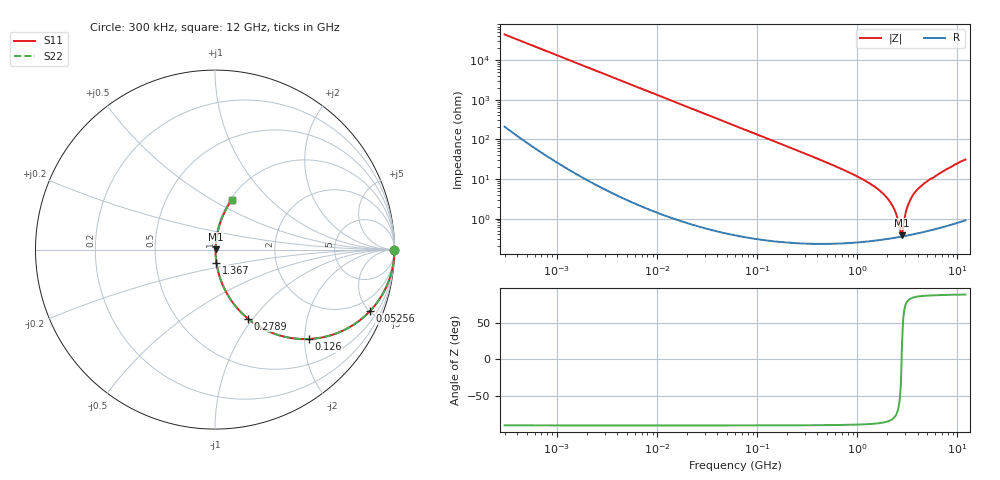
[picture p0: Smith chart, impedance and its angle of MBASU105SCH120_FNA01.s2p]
! MBASU105SCH120_FNA01  S-PARAMETER MODEL  ( General Type )
! Model Generated by TAIYO YUDEN Corporation (http://www.ty-top.com)
! Version 1.0
! TAIYO YUDEN Control No. 130207
! Copyright(c) 2013 TAIYO YUDEN CO.,LTD. All Rights Reserved.
! Product Description (link to TY-COMPAS)
! https://ds.yuden.co.jp/TYCOMPAS/or/detail?pn=MBASU105SCH120JFNA01&u=M
! Products Name : Multilayer Ceramic Capacitors
! Characteristics :
!  Capacitance : 12 pF , Rated Voltage : 50V , TCC : CH / C0H
!  Case Size : 1.0 x 0.5 / 0.039 x 0.02 [mm/inch] , Thickness : 0.5 / 0.02 [mm/inch]
!  (Conditions: Temperature = 25 degC , DC Bias Current/Voltage = 0A / 0V)
! External Node Assignments :
!  1  o---| |---o  2
! GND o---------o GND
! Frequency Range : 300000Hz  -  12GHz  [ 401 STEP ]
# MHz S RI R 50
! Freq[MHz].  S11 Real  S11 Imag  S21 Real  S21 Imag  S12 Real  S12 Imag  S22 Real  S22 Imag
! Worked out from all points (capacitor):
!   401 points, 300 kHz to 12 GHz, reference 50 ohm
!   read as one part in series: C = 12 pF near 316.3 kHz
!   lowest |Z| = 382 mohm at 2.795 GHz (marker M1)
!   series resonance near 2.768 GHz, so ESL is about 280 pH
!   S11 on the Smith chart (normalised r, x): 300 kHz: open; 52.56 MHz: 1.01, -5.05; 126 MHz: 1.01, -2.10; 278.9 MHz: 1.00, -0.94; 1.367 GHz: 1.01, -0.15; 12 GHz: 1.02, +0.62
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0.3  1 -0.00226  1.57e-05 0.00226  1.57e-05 0.00226  1 -0.00226
1.769972  0.9998 -0.0133  0.000197 0.0133  0.000197 0.0133  0.9998 -0.0133
10.44266  0.9938 -0.0782  0.00623 0.0782  0.00623 0.0782  0.9938 -0.0782
27.82928  0.9577 -0.2007  0.0423 0.2007  0.0423 0.2007  0.9577 -0.2007
52.55639  0.864 -0.342  0.136 0.342  0.136 0.342  0.864 -0.342
60  0.8298 -0.3749  0.1702 0.3749  0.1702 0.3749  0.8298 -0.3749
125.9782  0.5251 -0.498  0.4749 0.498  0.4749 0.498  0.5251 -0.498
278.9009  0.1829 -0.3841  0.8171 0.3841  0.8171 0.3841  0.1829 -0.3841
353.9943  0.1214 -0.3234  0.8786 0.3234  0.8786 0.3234  0.1214 -0.3234
783.7017  0.026 -0.1516  0.974 0.1516  0.974 0.1516  0.026 -0.1516
1366.97  0.00807 -0.073  0.9919 0.073  0.9919 0.073  0.00807 -0.073
1735.023  0.00508 -0.0465  0.9949 0.0465  0.9949 0.0465  0.00508 -0.0465
2088.533  0.00388 -0.0277  0.9961 0.0277  0.9961 0.0277  0.00388 -0.0277
2384.334  0.0035 -0.0149  0.9965 0.0149  0.9965 0.0149  0.0035 -0.0149
2650.866  0.00346 -0.00487  0.9965 0.00487  0.9965 0.00487  0.00346 -0.00487
2795.104  0.00352 0.00144  0.9965 -0.00144  0.9965 -0.00144  0.00352 0.00144
2870.14  0.00359 0.00515  0.9964 -0.00515  0.9964 -0.00515  0.00359 0.00515
3107.553  0.00399 0.0169  0.996 -0.0169  0.996 -0.0169  0.00399 0.0169
3276.641  0.0044 0.0245  0.9956 -0.0245  0.9956 -0.0245  0.0044 0.0245
3944.255  0.00697 0.0525  0.993 -0.0525  0.993 -0.0525  0.00697 0.0525
6879.757  0.0265 0.1416  0.9735 -0.1416  0.9735 -0.1416  0.0265 0.1416
12000  0.0937 0.2772  0.9063 -0.2772  0.9063 -0.2772  0.0937 0.2772
